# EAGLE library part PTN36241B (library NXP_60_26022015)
PLEASE CHECK AOUT+ AND AOUT- PTN36241B is a USB 3.0 (SuperSpeed) re-driver that enhances signal quality by performing receive equalization on the deteriorated input signal followed by transmit de-emphasis maximizing system link performance. With its superior differential signal conditioning and enhancement capability, the device delivers significant flexibility and performance scaling for various systems with different PCB trace and cable channel conditions and still benefit from optimum power consumption. PTN36241B is a dual-channel (channel A and channel B) device that supports data signaling rate of 5 Gbit/s through each channel. PTN36241B is flexibly powered from 3.3 V and is available in HVQFN24 4 mm × 4 mm package with 0.5 mm pitch. AAL Eindhoven MK
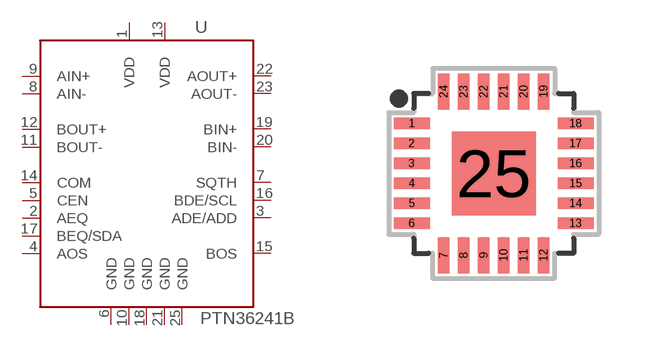
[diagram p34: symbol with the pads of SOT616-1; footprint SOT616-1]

Designator prefix U

## PTN36241B  [SOT616-1]
1  VDD  pwr
2  AEQ  in
3  ADE/ADD  in
4  AOS  in
5  CEN  in
6  GND  pwr
7  SQTH  in
8  AIN-  in
9  AIN+  in
10  GND  pwr
11  BOUT-  out
12  BOUT+  out
13  VDD  pwr
14  COM  in
15  BOS  in
16  BDE/SCL  in
17  BEQ/SDA  in
18  GND  pwr
19  BIN+  in
20  BIN-  in
21  GND  pwr
22  AOUT+  out
23  AOUT-  out
25  GND  pwr

## Footprint SOT616-1 (pad centres in mm)
SOT616-1 HVQFN24: plastic thermal enhanced very thin quad flat package; no leads; 24 terminals; body 4 x 4 x 0.85 mm JEDEC: MO-220 IEC: -- JEITA: --
smd 0.9 x 0.29: 1 -2.05,1.25; 2 -2.05,0.75; 3 -2.05,0.25; 4 -2.05,-0.25; 5 -2.05,-0.75; 6 -2.05,-1.25; 13 2.05,-1.25; 14 2.05,-0.75; 15 2.05,-0.25; 16 2.05,0.25; 17 2.05,0.75; 18 2.05,1.25
smd 0.29 x 0.9: 7 -1.25,-2.05; 8 -0.75,-2.05; 9 -0.25,-2.05; 10 0.25,-2.05; 11 0.75,-2.05; 12 1.25,-2.05; 19 1.25,2.05; 20 0.75,2.05; 21 0.25,2.05; 22 -0.25,2.05; 23 -0.75,2.05; 24 -1.25,2.05
smd 2.1 x 2.1: 25 0,0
